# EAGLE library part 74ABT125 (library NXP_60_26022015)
Quad bus BUFFER, 3-state The 74ABT125 high-performance BiCMOS device combines low static and dynamic power dissipation with high speed and high output drive. The 74ABT125 device is a quad buffer that is ideal for driving bus lines. The device features four Output Enables (1OE, 2OE, 3OE, 4OE), each controlling one of the 3-state outputs. AAL Eindhoven MK
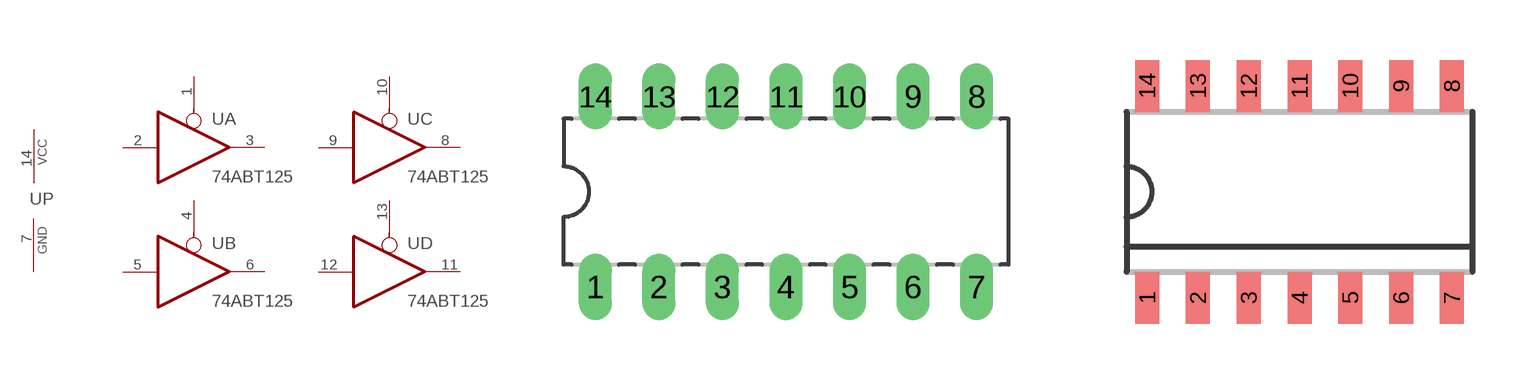
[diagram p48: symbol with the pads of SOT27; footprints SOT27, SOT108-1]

Designator prefix U; gates A=74125 B=74125 C=74125 D=74125 P=PWRN-1

## 74ABT125N  [SOT27]
1  A:OE  in
2  A:I  in
3  A:O  hiz
4  B:OE  in
5  B:I  in
6  B:O  hiz
7  P:GND  pwr
8  C:O  hiz
9  C:I  in
10  C:OE  in
11  D:O  hiz
12  D:I  in
13  D:OE  in
14  P:VCC  pwr

## 74ABT125D  [SOT108-1]
Pads as for SOT27

## 74ABT125DB  [SOT337]
Pads as for SOT27

## 74ABT125PW  [SOT402-1]
Pads as for SOT27

## 74ABT125BQ  [SOT762-1]
Pads as for SOT27

## Footprint SOT27 (pad centres in mm)
Dual In Line Package
drill 0.813 long: 1 -7.62,-3.81; 2 -5.08,-3.81; 3 -2.54,-3.81; 4 0,-3.81; 5 2.54,-3.81; 6 5.08,-3.81; 7 7.62,-3.81; 8 7.62,3.81; 9 5.08,3.81; 10 2.54,3.81; 11 0,3.81; 12 -2.54,3.81; 13 -5.08,3.81; 14 -7.62,3.81

## Footprint SOT108-1 (pad centres in mm)
SOT108-1 SO14: plastic small outline package; 14 leads; body width 3.9 mm; body thickness 1.47 mm JEDEC: MS-012 IEC: --
smd 0.6 x 1.3: 1 -3.81,-2.65; 2 -2.54,-2.65; 3 -1.27,-2.65; 4 0,-2.65; 5 1.27,-2.65; 6 2.54,-2.65; 7 3.81,-2.65; 8 3.81,2.65; 9 2.54,2.65; 10 1.27,2.65; 11 0,2.65; 12 -1.27,2.65; 13 -2.54,2.65; 14 -3.81,2.65

## Footprint SOT337 (pad centres in mm)
SOT337 SSOP14: plastic shrink small outline package; 14 leads; body width 5.3 mm JEDEC: MO-150 IEC: --
smd 0.4 x 1.2: 1 -1.95,-3.45; 2 -1.3,-3.45; 3 -0.65,-3.45; 4 0,-3.45; 5 0.65,-3.45; 6 1.3,-3.45; 7 1.95,-3.45; 8 1.95,3.45; 9 1.3,3.45; 10 0.65,3.45; 11 0,3.45; 12 -0.65,3.45; 13 -1.3,3.45; 14 -1.95,3.45

## Footprint SOT402-1 (pad centres in mm)
SOT402-1 TSSOP14: plastic thin shrink small outline package; 14 leads; body width 4.4 mm JEDEC: MO-153 IEC: ---
smd 0.6 x 1.35: 1 -2.05,-2.925; 7 2.05,-2.925; 8 2.05,2.925; 14 -2.05,2.925
smd 0.4 x 1.35: 2 -1.3,-2.925; 3 -0.65,-2.925; 4 0,-2.925; 5 0.65,-2.925; 6 1.3,-2.925; 9 1.3,2.925; 10 0.65,2.925; 11 0,2.925; 12 -0.65,2.925; 13 -1.3,2.925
